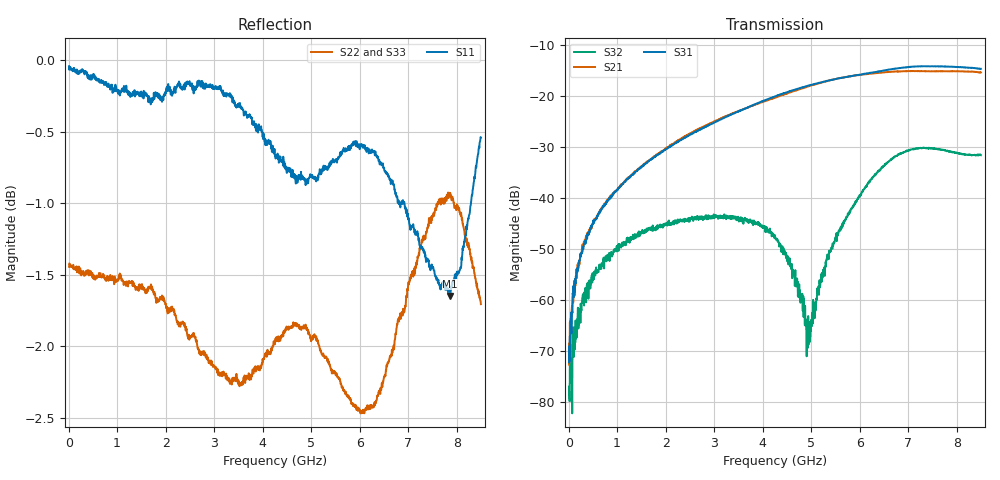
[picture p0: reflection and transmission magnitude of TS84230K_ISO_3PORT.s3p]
! Created with skrf (http://scikit-rf.org).
# Hz S RI R 50.0
!freq ReS11 ImS11 ReS12 ImS12 ReS13 ImS13
! ReS21 ImS21 ReS22 ImS22 ReS23 ImS23
! ReS31 ImS31 ReS32 ImS32 ReS33 ImS33
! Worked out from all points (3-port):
!   1601 points, 10 MHz to 8.5 GHz, reference 50 ohm
!   strongest paths, dB at 10 MHz, 2.132 GHz, 4.255 GHz, 6.378 GHz, 8.5 GHz:
!     S31: -69.3, -29.6, -20.0, -15.1, -14.6
!     S21: -72.7, -29.5, -20.3, -15.4, -15.3
!     S32: -77.0, -45.0, -47.3, -34.7, -31.6
!   lowest |S11| = -1.6 dB at 7.869 GHz (marker M1), VSWR 10.57, Z = 5.59 + j21.2 ohm
!   |S11| at or under -10 dB: nowhere
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1e7  0.9952 -0.0093  0.000157 9.78e-05  8.84e-05 -2.37e-05
     0.000139 0.000185  -0.8467 0.0048  -0.000172 -4.96e-06
     0.000311 0.000145  0.000137 -3.53e-05  -0.8501 0.00352
2.01025e8  0.9838 -0.1115  0.000187 0.00221  0.000195 0.00233
           0.000214 0.00222  -0.8425 0.0711  0.000155 0.000802
           5.25e-05 0.00207  -3.32e-05 0.000524  -0.8451 0.0681
7.210375e8  0.9059 -0.3792  -9.36e-05 0.00849  0.000237 0.00851
            0.000122 0.00845  -0.8042 0.2419  0.000507 0.00233
            -1.26e-05 0.00821  0.000704 0.00251  -0.806 0.2383
2.461488e9  0.2955 -0.9359  0.0107 0.0405  0.0103 0.0396
            0.0108 0.0405  -0.4227 0.6783  0.00514 0.00312
            0.0104 0.0392  0.00511 0.00357  -0.4372 0.6815
4.255e9  -0.349 -0.8574  0.0757 0.0606  0.0761 0.0644
         0.0755 0.0608  0.3976 0.6905  0.00355 -0.00215
         0.0764 0.0644  0.00382 -0.00202  0.3503 0.7013
4.9342e9  -0.5991 -0.6811  0.1162 0.0457  0.1178 0.0466
          0.1162 0.0458  0.6236 0.5088  -0.000131 -0.000372
          0.1181 0.0468  -0.000335 -0.000157  0.6283 0.4919
5.3587e9  -0.7779 -0.4853  0.1407 0.0218  0.1409 0.0233
          0.1409 0.0222  0.6944 0.3643  -0.0022 0.00139
          0.141 0.0233  -0.00204 0.00147  0.7079 0.3592
6.128106e9  -0.9311 -0.0254  0.1589 -0.0445  0.1628 -0.0357
            0.1586 -0.044  0.7552 0.0113  -0.00627 0.0111
            0.163 -0.0357  -0.00642 0.0111  0.7613 0.1253
7.868556e9  -0.57 0.5993  0.0674 -0.163  0.0728 -0.1812
            0.0674 -0.1625  0.3952 -0.8071  0.0264 0.0118
            0.0731 -0.1809  0.0262 0.0116  0.3613 -0.8123
8.5e9  -0.1405 0.9291  0.00821 -0.1715  0.00764 -0.1859
       0.00925 -0.1711  0.2304 -0.7887  0.0259 0.00673
       0.00824 -0.1858  0.0255 0.00711  0.2425 -0.7944
